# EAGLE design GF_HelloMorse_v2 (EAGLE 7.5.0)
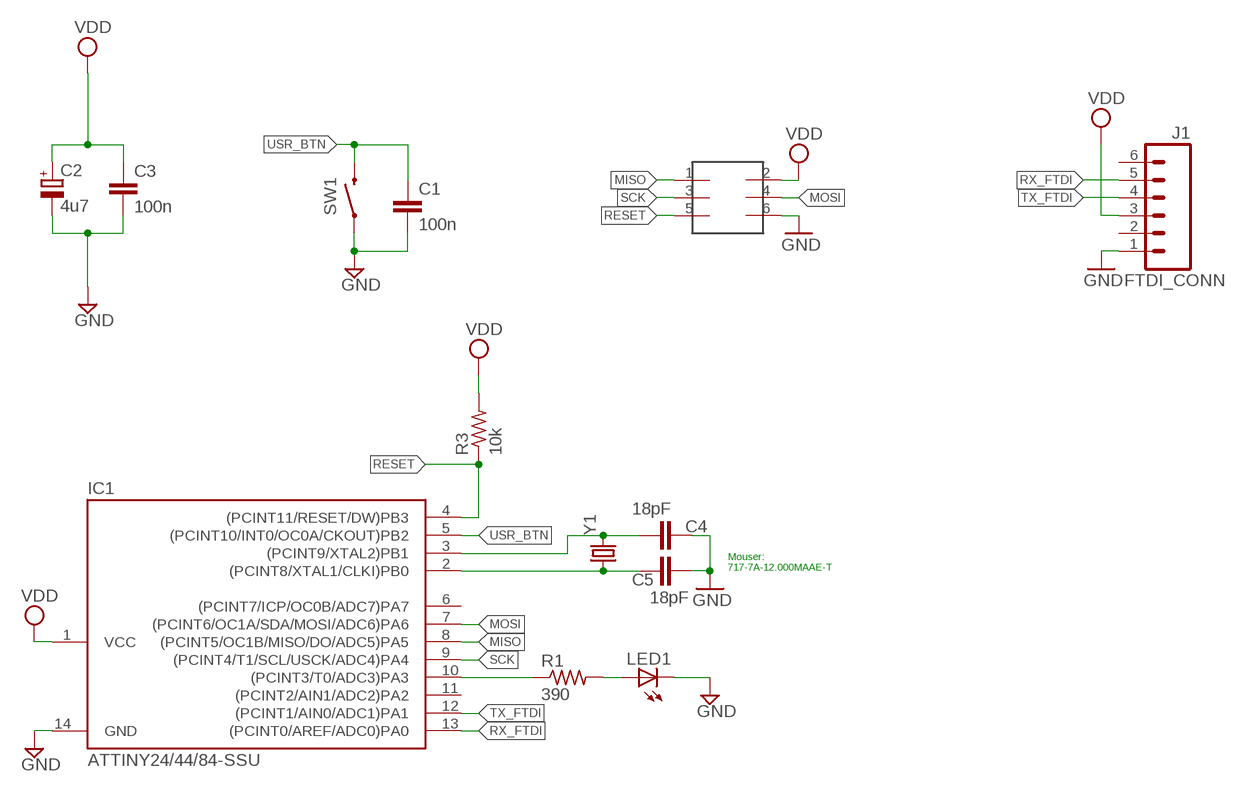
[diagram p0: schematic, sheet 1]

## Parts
C1  100n  C-EUC0603  [C0603]
C2  4u7  CPOL-EUSMCA  [SMC_A]
C3  100n  C-EUC0603  [C0603]
C4  18pF  C-EUC0603K  [C0603K]
C5  18pF  C-EUC0603K  [C0603K]
IC1  ATTINY24/44/84-SSU  [SOIC14]
ISP  2X3HEADER  [2X3_SMD]
J1  FTDI_CONN  M06SMD  [1X06-SMD]
LED1  LEDCHIPLED_1206  [CHIPLED_1206]
R1  390  R-US_R1206  [R1206]
R3  10k  R-US_R0603  [R0603]
SW1  SWITCH2  [TACTILE-SWITCH-1101NE]
Y1  CRYSTALTXC-7A  [CRYSTAL-TXC-7A]

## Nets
GND: C1.2 C2.- C3.2 C4.2 C5.2 IC1.14(GND) ISP.6 J1.1 LED1.C SW1.P$1
MISO: IC1.8((PCINT5/OC1B/MISO/DO/ADC5)PA5) ISP.1
MOSI: IC1.7((PCINT6/OC1A/SDA/MOSI/ADC6)PA6) ISP.4
N$1: IC1.10((PCINT3/T0/ADC3)PA3) R1.1
N$2: LED1.A R1.2
N$3: C5.1 IC1.2((PCINT8/XTAL1/CLKI)PB0) Y1.P$1
N$7: C4.1 IC1.3((PCINT9/XTAL2)PB1) Y1.P$2
RESET: IC1.4((PCINT11/RESET/DW)PB3) ISP.5 R3.1
RX_FTDI: IC1.13((PCINT0/AREF/ADC0)PA0) J1.5
SCK: IC1.9((PCINT4/T1/SCL/USCK/ADC4)PA4) ISP.3
TX_FTDI: IC1.12((PCINT1/AIN0/ADC1)PA1) J1.4
USR_BTN: C1.1 IC1.5((PCINT10/INT0/OC0A/CKOUT)PB2) SW1.P$2
VDD: C2.+ C3.1 IC1.1(VCC) ISP.2 J1.3 R3.2
Unconnected: IC1.6((PCINT7/ICP/OC0B/ADC7)PA7) IC1.11((PCINT2/AIN1/ADC2)PA2) J1.2 J1.6

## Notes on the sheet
- Mouser:
  717-7A-12.000MAAE-T

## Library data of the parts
C1 C3-C5 = rcl:C-EU: CAPACITOR, European symbol
C2 = rcl:CPOL-EU: POLARIZED CAPACITOR, European symbol
IC1 = attiny24_44_84:ATTINY24/44/84
ISP = mellis:2X3HEADER
J1 = SparkFun-Connectors:M06: Header 6 Standard 6-pin 0.1" header. Use with straight break away headers (SKU : PRT-00116), right angle break away headers (PRT-00553), swiss pins (PRT-00743), machine pins (PRT-00117), and female headers (PRT-00115). Molex polarized connector foot print use with SKU : PRT-08094 with associated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; PROD_ID: CONN-08971; VALUE: RA 6Pin SMD
LED1 = led:LED: LED
R1 R3 = rcl:R-US_: RESISTOR, American symbol
SW1 = SparkFun-Electromechanical:SWITCH2
Y1 = SparkFun-FreqCtrl:CRYSTAL: Various standard crystals. Proven footprints. Spark Fun Electronics SKU : COM-00534

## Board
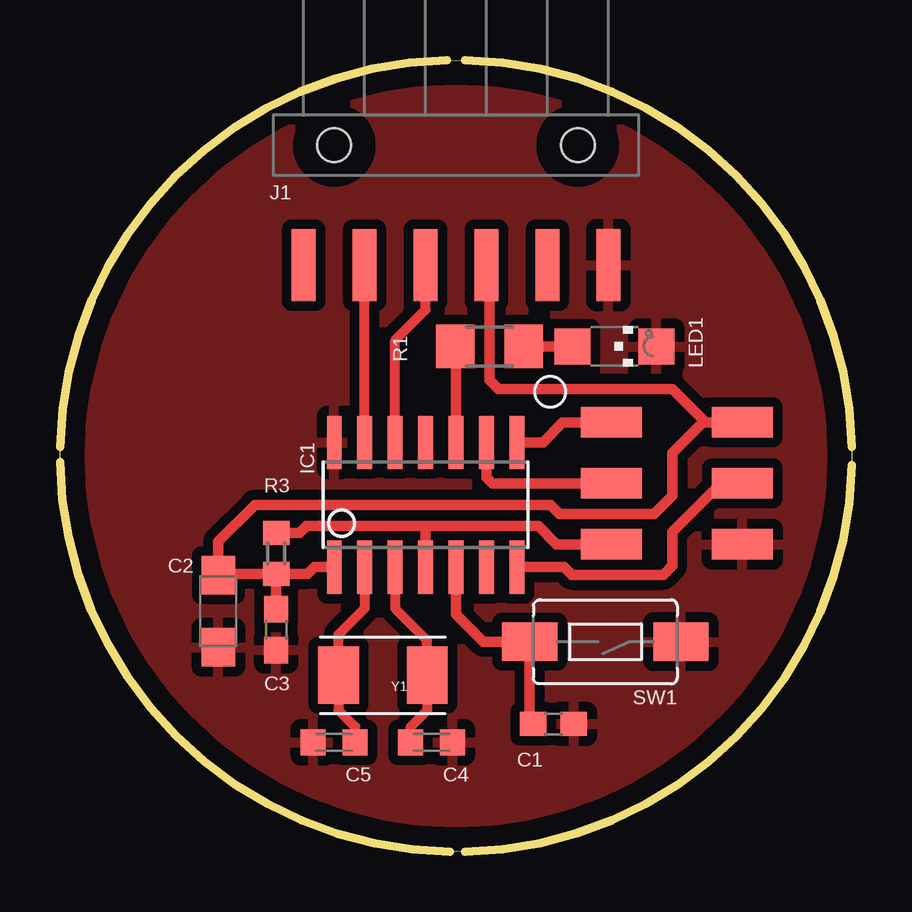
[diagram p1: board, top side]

Size 33.02 x 33.02 mm. Coordinates in mm from the lower left corner, seen from the top.
Outline: 0,16.51 arc-180 33.02,16.51 arc-180 0,16.51
Copper layers (1*16): Top 0.035mm / dielectric 1.5mm / Bottom 0.035mm
Design rules "default *": minimum track width 10mil, minimum drill 24mil, track to track 16mil, track to pad 16mil, pad to pad 16mil, via to via 16mil, smd to smd 16mil, copper to edge 40mil, drill to drill 8mil, minimum pad ring 10mil, minimum via ring 8mil, stop-mask expansion 4mil, vias tented up to drill 0mil, thermal gap 17mil
Milling: 4 lines

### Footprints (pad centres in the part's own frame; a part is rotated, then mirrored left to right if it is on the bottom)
C0603 = smd 1.1 x 1: 1 -0.85,0; 2 0.85,0
SMC_A = smd 1.6 x 1.4: + -1.5,0; - 1.5,0
C0603K = smd 1.05 x 1.08: 1 -0.875,0; 2 0.875,0
SOIC14 = smd 0.61 x 2.21: 1 -3.81,-2.603; 2 -2.54,-2.603; 3 -1.27,-2.603; 4 0,-2.603; 5 1.27,-2.603; 6 2.54,-2.603; 7 3.81,-2.603; 8 3.81,2.603; 9 2.54,2.603; 10 1.27,2.603; 11 0,2.603; 12 -1.27,2.603; 13 -2.54,2.603; 14 -3.81,2.603
2X3_SMD = smd 2.54 x 1.27: 1 -2.54,2.54; 2 2.92,2.54; 3 -2.54,0; 4 2.92,0; 5 -2.54,-2.54; 6 2.92,-2.54
1X06-SMD = smd 1 x 3: 1 -6.35,5; 2 -3.81,5; 3 -1.27,5; 4 1.27,5; 5 3.81,5; 6 6.35,5 | hole 1.4: -5.08,0; 5.08,0
CHIPLED_1206 = smd 1.5 x 1.5: A 0,-1.75; C 0,1.75
R1206 = smd 1.6 x 1.803: 1 -1.422,0; 2 1.422,0
R0603 = smd 1 x 1.1: 1 -0.85,0; 2 0.85,0
TACTILE-SWITCH-1101NE = smd 2.3 x 1.6: P$1 -3.15,0; P$2 3.15,0
CRYSTAL-TXC-7A = smd 1.7 x 2.4: P$1 1.85,0; P$2 -1.85,0

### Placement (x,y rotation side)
C1  20.57,5.33 0 top
C2  6.6,10.03 270 top
C3  9.02,9.27 270 top
C4  15.49,4.57 0 top
C5  11.43,4.57 180 top
IC1  15.24,14.48 0 top
ISP  25.53,15.37 0 top
J1  16.51,29.46 180 top
LED1  23.11,21.08 270 top
R1  17.91,21.08 0 top
R3  9.02,12.45 270 top
SW1  22.73,8.76 180 top
Y1  13.46,7.37 180 top

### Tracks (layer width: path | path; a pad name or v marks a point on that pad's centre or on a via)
GND
  pour Top (isolate 0.406): 0,0 33.02,0 33.02,33.02 0,33.02
MISO
  Top 0.432: IC1.8 20.13,17.08 20.95,17.91 ISP.1
MOSI
  Top 0.432: IC1.7 21.02,11.87 21.34,11.56 25.15,11.56 25.53,11.94 25.53,13.34 27.56,15.37 ISP.4
N$1
  Top 0.432: IC1.10 16.51,21.06 R1.1
N$2
  Top 0.432: R1.2 LED1.A
N$3
  Top 0.406: C5.1 12.3,5.22 11.61,5.91 Y1.P$1 11.61,9.07 12.7,10.16 IC1.2
N$7
  Top 0.406: C4.1 14.62,5.22 15.31,5.91 Y1.P$2 15.31,8.82 13.97,10.16 IC1.3
RESET
  Top 0.432: 15.24,13.59 19.94,13.59 20.7,12.83 ISP.5 | IC1.4 15.24,13.59 | R3.1 9.99,13.3 10.29,13.59 15.24,13.59
RX_FTDI
  Top 0.406: IC1.13 J1.5
SCK
  Top 0.432: IC1.9 17.78,15.62 18.03,15.37 ISP.3
TX_FTDI
  Top 0.406: IC1.12 13.97,21.34 15.24,22.61 J1.4
USR_BTN
  Top 0.432: IC1.5 16.51,9.91 17.65,8.76 SW1.P$2 19.58,5.38 C1.1
VDD
  Top 0.432: ISP.2 26.92,17.91 | 26.92,17.91 26.8,17.91 25.53,16.64 25.53,14.86 24.77,14.1 20.83,14.1 20.45,14.48 8.13,14.48 6.6,12.95 C2.+ 6.67,11.6 R3.2 | IC1.1 10.6,11.87 10.33,11.6 R3.2 | R3.2 C3.1 | 26.92,17.91 25.53,19.3 18.29,19.3 17.91,19.68 17.91,24.34 J1.3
